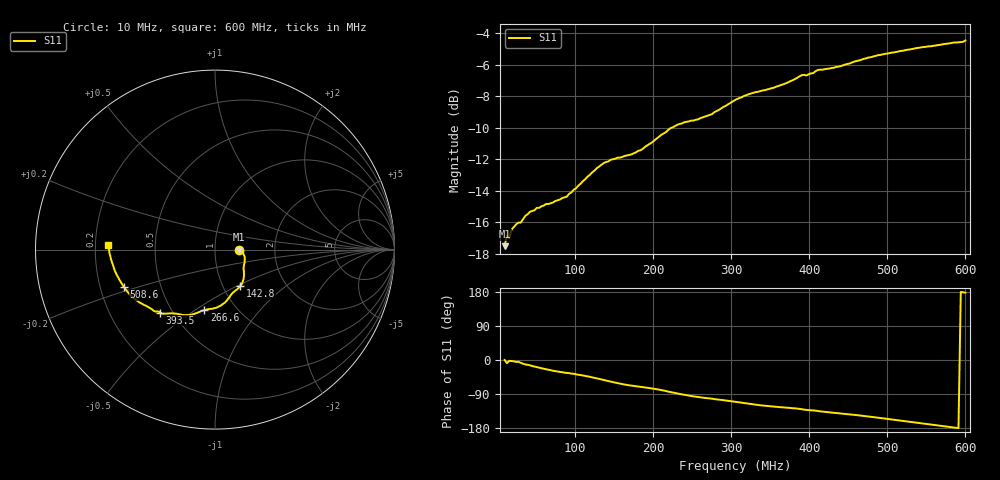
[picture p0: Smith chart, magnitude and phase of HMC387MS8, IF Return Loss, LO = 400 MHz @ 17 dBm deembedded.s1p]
!Hittite Microwave Corporation
!12 Elizabeth Drive
!Chelmsford, MA 01824
!Tel: 978-250-3343
!Fax: 978-250-3373
!Device: HMC387MS8, 450-500 MHz, GaAs MMIC High IP3 Mixer in 8-lead plastic SMT package
!Misc: IF Return Loss, LO = 400 MHz @ 17 dBm, Room
# MHZ S MA R 50
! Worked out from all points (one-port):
!   201 points, 10 MHz to 600 MHz, reference 50 ohm
!   lowest |S11| = -17.5 dB at 10 MHz (marker M1), VSWR 1.31, Z = 65.3 + j0.0463 ohm
!   |S11| at or under -10 dB: start of sweep to 224.2 MHz
!   S11 on the Smith chart (normalised r, x): 10 MHz: 1.31, +0.00; 142.8 MHz: 1.20, -0.52; 266.6 MHz: 0.71, -0.55; 393.5 MHz: 0.43, -0.38; 508.6 MHz: 0.30, -0.18; 600 MHz: 0.25, +0.02
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10  0.133 0.1
12.95  0.144 -8.4
15.9  0.141 -2.2
18.85  0.15 -2.7
27.7  0.158 -4.7
30.65  0.158 -7.4
42.45  0.171 -13.9
83.75  0.189 -32.2
89.65  0.191 -34.1
122.1  0.228 -45.7
136.85  0.244 -52.7
142.75  0.247 -55.7
157.5  0.254 -62.0
184.05  0.268 -70.8
204.7  0.292 -77.1
231.25  0.323 -88.3
266.65  0.343 -100.1
305  0.387 -110.2
337.45  0.413 -119.6
378.75  0.447 -127.1
393.5  0.465 -131.1
408.25  0.478 -133.7
452.5  0.506 -143.4
482  0.532 -150.7
508.55  0.548 -157.7
526.25  0.559 -162.7
552.8  0.573 -169.6
600  0.598 177.7
